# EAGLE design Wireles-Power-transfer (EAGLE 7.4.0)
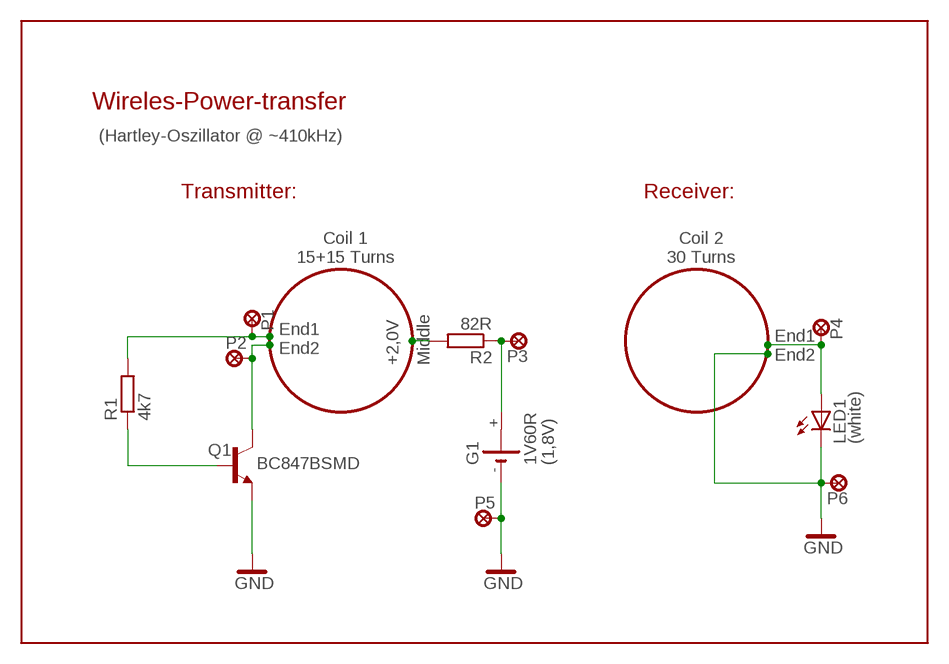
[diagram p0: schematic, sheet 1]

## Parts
G1  1V60R  [1V60R]
LED1  (white)  LEDSML0805  [SML0805]
P1  LSP13  [LSP13]
P2  LSP13  [LSP13]
P3  LSP13  [LSP13]
P4  LSP13  [LSP13]
P5  LSP13  [LSP13]
P6  LSP13  [LSP13]
Q1  BC847BSMD  [SOT23]
R1  4k7  R-EU_R0603  [R0603]
R2  82R  R-EU_R0603  [R0603]

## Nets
GND: G1.- LED1.C P5.P$1(MP) P6.P$1(MP) Q1.2(E)
N$1: Q1.1(B) R1.1
N$2: P2.P$1(MP) Q1.3(C)
N$3: P1.P$1(MP) R1.2
N$4: G1.+ P3.P$1(MP) R2.1
N$5: R2.2
N$6: LED1.A P4.P$1(MP)
Unconnected: G1.+@1(+)

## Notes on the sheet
- Wireles-Power-transfer
- (Hartley-Oszillator @ ~410kHz)
- Transmitter: | Receiver:
- Coil 1
  15+15 Turns
- Coil 2
  30 Turns
- End1
  End2
- End1
  End2
- +2,0V | Middle
- (1,8V)

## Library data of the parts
G1 = battery:1V60R: NC ACCU Varta
LED1 = led:LED: LED
P1-P6 = solpad-smd:LSP13: SMD Solder-Pad
Q1 = transistor-npn:BC847*: NPN Transistor
R1 R2 = rcl1:R-EU_: RESISTOR, European symbol

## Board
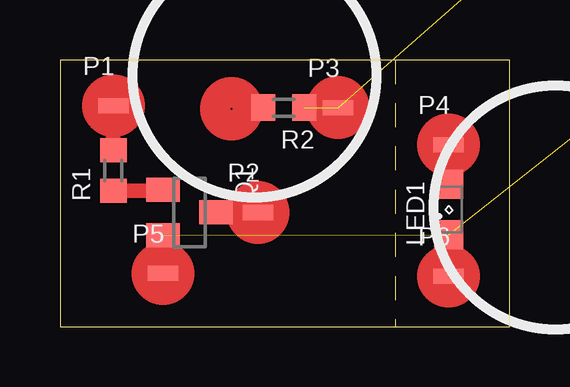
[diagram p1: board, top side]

Size 18.73 x 11.11 mm. Coordinates in mm from the lower left corner, seen from the top.
Outline: 13.97,0 0,0 0,11.11 13.97,11.11
Outline: 13.97,0 18.73,0 18.73,11.11 13.97,11.11
Outline: 13.97,11.11 13.97,0
Copper layers (1*16): Top 0.035mm / dielectric 1.5mm / Bottom 0.035mm
Design rules "default": minimum track width 10mil, minimum drill 24mil, track to track 8mil, track to pad 8mil, pad to pad 8mil, via to via 8mil, smd to smd 8mil, copper to edge 40mil, drill to drill 8mil, minimum pad ring 10mil, minimum via ring 8mil, stop-mask expansion 4mil, vias tented up to drill 0mil, thermal gap 10mil

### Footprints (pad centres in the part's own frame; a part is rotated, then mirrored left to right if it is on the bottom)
1V60R = drill 1.321 pad 3.15 octagon: + -2.54,-5.08; +@1 -2.54,5.08; - 3.683,0
SML0805 = smd 1.2 x 1.2: A 1.05,0; C -1.05,0
LSP13 = smd 1.27 x 0.635: P$1 0,0
SOT23 = smd 1 x 1.4: 1 -0.95,-1.1; 2 0.95,-1.1; 3 0,1.1
R0603 = smd 1 x 1.1: 1 -0.85,0; 2 0.85,0

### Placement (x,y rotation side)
G1  not placed on the board
LED1  16.19,4.88 90 top
P1  2.22,9.21 0 top
P2  8.26,4.76 0 top
P3  11.59,9.13 0 top
P4  16.19,7.58 0 top
P5  4.29,2.22 0 top
P6  16.19,2.1 0 top
Q1  5.4,4.76 270 top
R1  2.22,6.51 90 top
R2  9.33,9.13 180 top

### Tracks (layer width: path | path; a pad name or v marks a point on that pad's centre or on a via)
GND  (2 unrouted)
  Top 0.61: Q1.2 4.29,3.81 P5.P$1 | LED1.C P6.P$1
N$1
  Top 0.61: R1.1 4.3,5.66 Q1.1
N$2
  Top 0.61: Q1.3 P2.P$1
N$3
  Top 0.61: R1.2 P1.P$1
N$4  (2 unrouted)
N$6
  Top 0.61: LED1.A P4.P$1
(copper drawn outside any net)
  shapes: Top circle x1

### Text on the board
Document: GND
